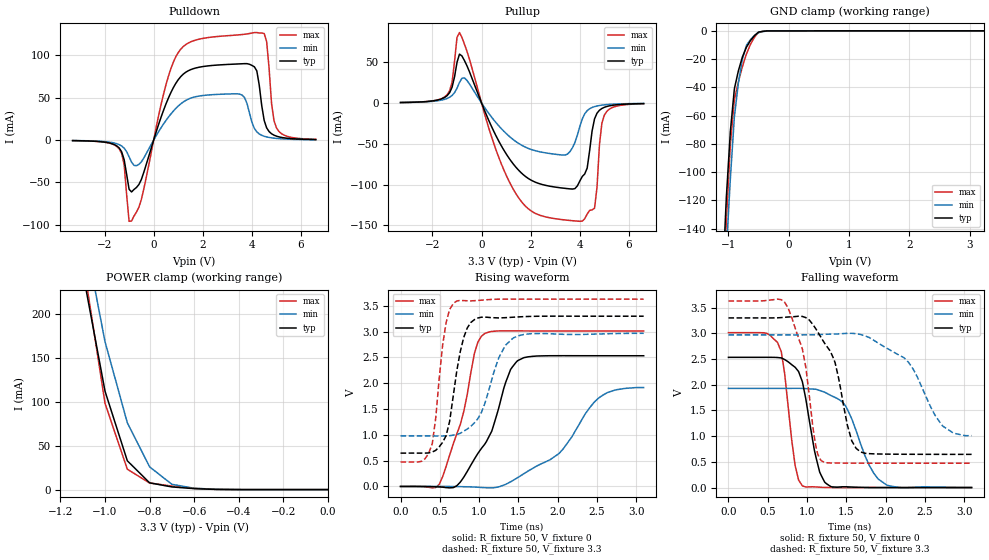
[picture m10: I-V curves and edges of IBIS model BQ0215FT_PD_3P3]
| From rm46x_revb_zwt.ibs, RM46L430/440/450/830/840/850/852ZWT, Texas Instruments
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|   Model Cell BQ0215FT_PD_3P3
|BQ0215FT_PD_3P3
[Model]   BQ0215FT_PD_3P3
Model_type   I/O
Polarity   Non-Inverting
Enable   Active-Low
Vinl =  1.15
Vinh =  1.55
Cref =  15.0001pF
Rref =  101.0000M
Vref =  0V
Vmeas =  1.65
C_comp   1.2p   1.2p   1.2p
[Model Spec]
Vinl   1.15   1.02   1.28
Vinh   1.55   1.45   1.65
[Temperature Range]   25   155   -40
[Voltage Range]   3.3   2.97   3.63
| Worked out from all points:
|   slope of the pulldown table from 0 to 0.495 V, typ, clamps not added: 11.7 ohm
|   slope of the pullup table from 0 to 0.495 V, typ, clamps not added: 14.3 ohm
|   GND clamp passes 1 mA (typ) near -0.50 V on its own axis
|   POWER clamp passes 1 mA (typ) near -0.59 V on its own axis
|   rising waveform, R_fixture 50, V_fixture 0: 20-80 % time 410ps typ, 692ps min, 296ps max; typ from 0 V to 2.53 V
|   rising waveform, R_fixture 50, V_fixture 3.3: 20-80 % time 174ps typ, 268ps min, 133ps max; typ from 0.646 V to 3.3 V
|   falling waveform, R_fixture 50, V_fixture 0: 20-80 % time 182ps typ, 303ps min, 138ps max; typ from 2.53 V to 0 V
|   falling waveform, R_fixture 50, V_fixture 3.3: 20-80 % time 279ps typ, 461ps min, 209ps max; typ from 3.3 V to 0.646 V
[POWER_clamp]
|   voltage   I(typ)   I(min)   I(max)
-3.3V     4.034A     4.621A     4.844A
-1.1V     248.3mA    300.9mA    262.9mA
-1.067V   202.9mA    256.8mA    208mA
-1.033V   157.5mA    212.7mA    153.2mA
-1V       112.1mA    168.6mA    98.33mA
-900mV    32.89mA    76.22mA    23.26mA
-800mV    7.724mA    25.95mA    7.513mA
-700mV    3.052mA    6.046mA    4.029mA
-600mV    1.107mA    1.536mA    1.463mA
-500mV    206.8uA    377.5uA    241.6uA
0V        19.75uA    8.577uA    38.26uA
[Pulldown]
|   voltage   I(typ)   I(min)   I(max)
-3.3V     -583.8uA   -509.7uA   -562.9uA
-1.4V     -9.427mA   -5.344mA   -10.39mA
-1.2V     -23.28mA   -9.543mA   -29.38mA
-1V       -58.07mA   -19.65mA   -95.88mA
-900mV    -61.21mA   -25.99mA   -95.6mA
1V        71.34mA    40.23mA    103.4mA
3.5V      90.06mA    54.34mA    124.5mA
4.2V      81.77mA    9.741mA    127mA
4.6V      14.51mA    3.766mA    116.4mA
4.8V      7.515mA    2.688mA    43.16mA
5V        4.703mA    2.013mA    14.54mA
6.6V      667.2uA    491.6uA    918.8uA
[Pullup]
|   voltage   I(typ)   I(min)   I(max)
-3.3V     645.2uA    598.5uA    584.2uA
-1.4V     9.107mA    5.632mA    10.27mA
-900mV    59.97mA    25.19mA    86.39mA
600mV     -40.93mA   -24.45mA   -58.47mA
1.4V      -78.76mA   -47.33mA   -111.2mA
3.4V      -104.6mA   -63.8mA    -143.4mA
4V        -95.69mA   -28.77mA   -145mA
4.3V      -79.78mA   -9.339mA   -136mA
4.6V      -19.38mA   -4.395mA   -129mA
4.8V      -8.841mA   -3.032mA   -50.9mA
5V        -5.243mA   -2.22mA    -14.75mA
6.6V      -699.3uA   -541.6uA   -880.5uA
[GND_clamp]
|   voltage   I(typ)   I(min)   I(max)
-3.3V     -3.232A    -2.867A    -4.906A
-1.1V     -181.4mA   -214mA     -212mA
-1.033V   -118mA     -155.8mA   -134.9mA
-966.7mV  -71.19mA   -104.7mA   -80.42mA
-900mV    -40.99mA   -60.83mA   -48.65mA
-833.3mV  -28.24mA   -36.87mA   -36.02mA
-766.7mV  -18.43mA   -20.01mA   -25.25mA
-700mV    -11.56mA   -10.24mA   -16.33mA
-566.7mV  -3.321mA   -3.252mA   -4.457mA
-500mV    -890.7uA   -1.261mA   -1.032mA
-300mV    -7.986uA   -19.12uA   -10.93uA
3.233V    19.75uA    12.66uA    38.26uA
[Ramp]
| variable   typ   min   max
dV/dt_f   1.613181/0.2886499n   1.213001/0.4927531n   1.916018/0.2146928n
dV/dt_r   1.537132/0.4178036n   1.174403/0.7161375n   1.826024/0.2990962n
R_load = 50
[Rising Waveform]
R_fixture = 50
V_fixture = 0
V_fixture_min = 0
V_fixture_max = 0
|   time   V(typ)   V(min)   V(max)
0s        -1.079uV   -4.063uV   -946.9nV
492ps     -9.168mV   409.6uV    39.43mV
716ps     14.02mV    -2.645mV   1.023V
804ps     179mV      -5.209mV   1.453V
940ps     532.6mV    -11.53mV   2.581V
1.072ns   821.1mV    -23.64mV   2.965V
1.488ns   2.436V     169.6mV    3.015V
2.016ns   2.534V     639.8mV    3.014V
2.516ns   2.533V     1.71V      3.014V
3.092ns   2.533V     1.917V     3.014V
[Rising Waveform]
R_fixture = 50
V_fixture = 3.3
V_fixture_min = 2.97
V_fixture_max = 3.63
|   time   V(typ)   V(min)   V(max)
0s        646.4mV    979.9mV    473.7mV
268ps     645.9mV    980.1mV    487.4mV
404ps     667.7mV    979.5mV    830.9mV
580ps     984.8mV    979.6mV    3.178V
716ps     2.245V     1.006V     3.594V
892ps     3.175V     1.164V     3.597V
1.028ns   3.28V      1.433V     3.61V
1.248ns   3.266V     2.487V     3.629V
1.444ns   3.281V     2.885V     3.63V
3.092ns   3.3V       2.968V     3.63V
[Falling Waveform]
R_fixture = 50
V_fixture = 0
V_fixture_min = 0
V_fixture_max = 0
|   time   V(typ)   V(min)   V(max)
0s        2.533V     1.929V     3.014V
624ps     2.53V      1.929V     2.825V
716ps     2.489V     1.93V      2.203V
848ps     2.34V      1.93V      430.5mV
940ps     2.06V      1.929V     33.33mV
1.16ns    303.1mV    1.889V     7.582mV
1.292ns   28.83mV    1.799V     1.041mV
1.488ns   15.02mV    1.593V     271.1uV
2.016ns   549.3uV    45.61mV    224.6uV
3.092ns   285.6uV    1.424mV    30.84uV
[Falling Waveform]
R_fixture = 50
V_fixture = 3.3
V_fixture_min = 2.97
V_fixture_max = 3.63
|   time   V(typ)   V(min)   V(max)
0s        3.3V       2.97V      3.63V
760ps     3.318V     2.97V      3.488V
940ps     3.329V     2.97V      2.698V
1.092ns   3.131V     2.973V     981.1mV
1.18ns    2.915V     2.978V     523.2mV
1.356ns   2.43V      2.987V     478mV
1.68ns    692.6mV    2.978V     474.3mV
2.292ns   647.8mV    2.432V     473.9mV
2.724ns   646.4mV    1.198V     473.9mV
3.092ns   646.2mV    1.01V      473.8mV
